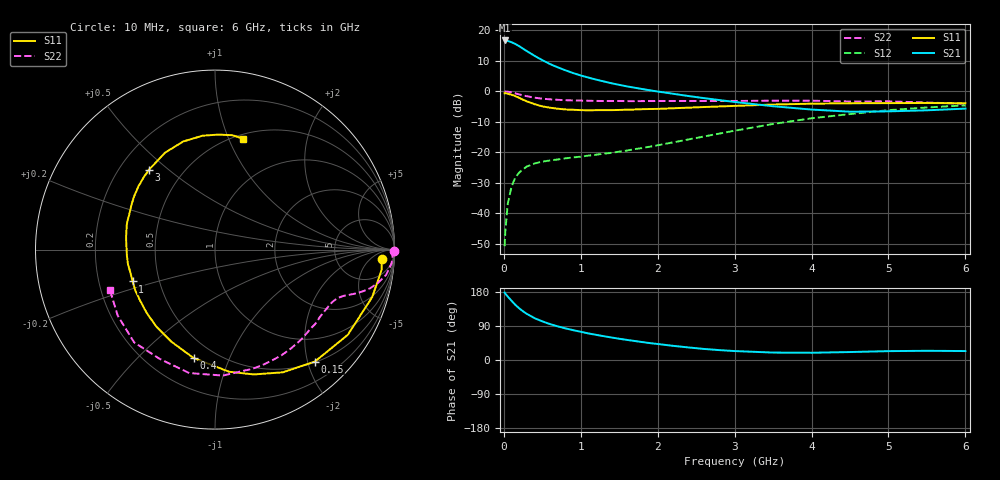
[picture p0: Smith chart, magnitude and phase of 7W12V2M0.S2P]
! Infineon Technologies  Discrete & RF Semiconductors
! BFS17W
! Si NPN RF Bipolar Junction Transistor in SOT323
! VCE = 12 V  IC = 2 mA
! Common Emitter S-Parameters:  August  1999
# GHz  S  MA  R  50
!  f  S11  S21  S12  S22
! GHz  MAG  ANG  MAG  ANG  MAG  ANG  MAG  ANG
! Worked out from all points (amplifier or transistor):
!   36 points, 10 MHz to 6 GHz, reference 50 ohm
!   highest |S21| = 16.7 dB at 10 MHz (marker M1)
!   |S21| within 3 dB of that: start of sweep to 268.6 MHz
!   unconditionally stable (mu >= 1): 872.6 MHz to 2.569 GHz; 4.906 GHz to end of sweep
!   at 250 MHz: K = 0.35, MSG = 19.7 dB, |S12| = -25.5 dB
!   at 1.4 GHz: K = 1.24, MAG = 8.4 dB, |S12| = -20.2 dB
!   at 6 GHz: K = 1.07, MAG = -2.1 dB, |S12| = -4.6 dB
!   S11 on the Smith chart (normalised r, x): 10 MHz: 17, -13; 150 MHz: 0.51, -2.13; 400 MHz: 0.38, -0.75; 1 GHz: 0.35, -0.16; 3 GHz: 0.32, +0.43; 6 GHz: 0.55, +1.13
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0.01  0.9299 -3.3  6.826 178.0  0.0029 84.3  0.9994 -0.4
0.02  0.9355 -6.8  6.793 175.1  0.0052 88.1  0.9899 -1.7
0.05  0.915 -16.8  6.716 167.6  0.0141 84.9  0.9872 -4.4
0.1  0.8792 -32.7  6.383 156.3  0.0276 73.5  0.9638 -8.4
0.15  0.8359 -48.3  5.981 145.4  0.0389 64.6  0.9272 -11.5
0.2  0.7816 -61.0  5.497 136.3  0.0467 59.8  0.8925 -13.9
0.25  0.7285 -72.7  5.002 128.4  0.053 54.6  0.8593 -15.6
0.3  0.6851 -83.4  4.558 121.6  0.0587 51.1  0.8316 -16.9
0.4  0.6156 -101.2  3.816 110.4  0.0657 46.3  0.7876 -18.7
0.5  0.5677 -115.4  3.248 101.9  0.0705 44.0  0.759 -19.9
0.6  0.5392 -127.3  2.803 94.8  0.0737 43.6  0.7399 -21.2
0.7  0.5194 -136.9  2.476 88.8  0.0765 44.2  0.7267 -22.5
0.8  0.5051 -145.6  2.215 83.5  0.0798 45.0  0.7165 -24.0
1  0.492 -158.9  1.821 74.5  0.0851 48.1  0.7059 -27.0
1.1  0.4886 -165.6  1.68 70.1  0.0885 49.3  0.701 -29.0
1.6  0.5006 171.7  1.207 53.0  0.107 59.0  0.6917 -39.0
2.2  0.528 151.9  0.913 37.4  0.1458 68.8  0.6947 -52.7
3  0.5775 129.5  0.67 23.6  0.2263 72.9  0.696 -72.6
3.5  0.6077 117.2  0.57 19.6  0.2921 70.7  0.7031 -86.5
4.5  0.6384 96.2  0.464 21.0  0.4243 59.2  0.6825 -116.7
5.5  0.6446 81.3  0.489 24.3  0.544 45.4  0.6551 -145.8
6  0.6372 75.6  0.521 23.6  0.5902 38.5  0.6272 -158.8
